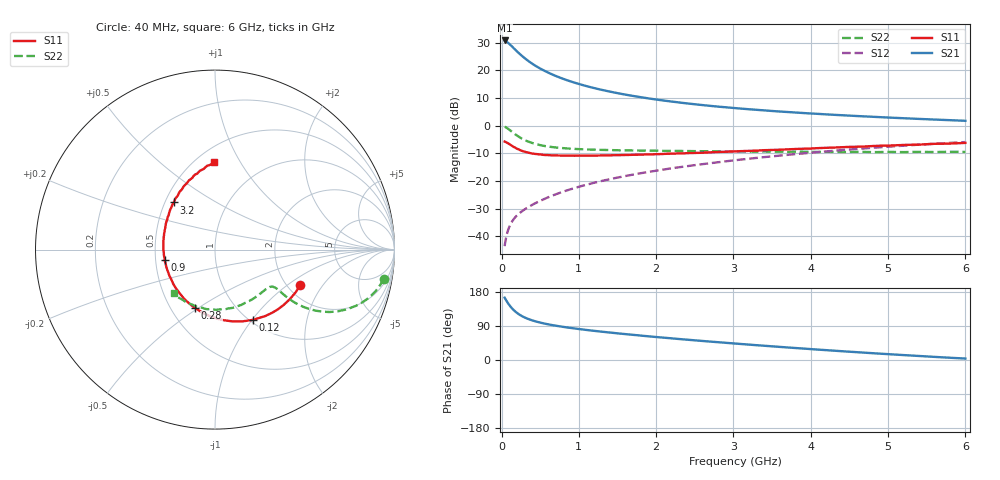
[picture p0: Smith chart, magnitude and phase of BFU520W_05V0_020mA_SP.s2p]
! Filename:  P:\Prog\Test\Noise\ATS_data\Testdata_Net\Run2\BFU520W_APM2013_06_A05_05p0V_020mA_SP_CM01_D.s2p
! Date/Time: Tue 26/Mar/2013 18:01:41
! BFU520W_APM2013_06_A05_05p0V_1to20mA_SP_CM01_Bias8_R.s2p
! MDIF S-parameter v. bias file
! BFU520W_APM2013_06_A05_05p0V_1to20mA_SP_CM01
! Date/time Thu Mar 21 14:22:37 2013
! VAR V_out= 5.0010
! VAR I_out= 19.9950
! VAR V_in= 0.8452
! VAR I_in= 0.2325
! Device data file deembeded for feedlines and parallel
! Original file: \Run2\BFU520W_APM2013_06_A05_05p0V_020mA_SP_CM01_R.s2p
! Feed-files: PR019V01_070313_Feed1.s2p, PR019V01_070313_Feed2.s2p
! Parallel-file: PR019V01_070313_Par.s2p
# MHz S MA R 50
!  Freq-MHz  S11-mag  S11-arg  S21-mag  S21-arg  S12-mag  S12-arg  S22-mag  S22-arg
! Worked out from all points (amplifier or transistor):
!   98 points, 40 MHz to 6 GHz, reference 50 ohm
!   highest |S21| = 30.8 dB at 40 MHz (marker M1)
!   |S21| within 3 dB of that: start of sweep to 164.9 MHz
!   unconditionally stable (mu >= 1): 975.5 MHz to 2.09 GHz
!   at 300 MHz: K = 0.71, MSG = 27.4 dB, |S12| = -30.3 dB
!   at 1.6 GHz: K = 1.01, MAG = 14.0 dB, |S12| = -18.3 dB
!   at 6 GHz: K = 0.84, MSG = 3.8 dB, |S12| = -5.9 dB
!   S11 on the Smith chart (normalised r, x): 40 MHz: 2.33, -1.26; 120 MHz: 1.04, -1.01; 280 MHz: 0.66, -0.49; 900 MHz: 0.56, -0.07; 3.2 GHz: 0.56, +0.33; 6 GHz: 0.61, +0.78
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40  0.5154 -22.7  34.82 164.6  0.006581 81.1  0.955 -9.9
50  0.5081 -28.1  34.44 161.0  0.008026 79.9  0.9415 -12.1
60  0.5002 -33.4  33.41 157.6  0.009551 78.1  0.925 -14.4
80  0.4831 -43.6  31.92 151.1  0.01223 75.0  0.8875 -18.4
100  0.4641 -52.8  30.16 145.3  0.01463 72.4  0.8456 -21.7
120  0.4451 -61.6  28.48 140.0  0.01681 70.4  0.8045 -24.5
160  0.4109 -76.6  25.04 131.3  0.02055 67.7  0.7273 -28.6
200  0.3831 -89.1  22.08 124.4  0.02372 66.3  0.6616 -31.0
240  0.3608 -99.7  19.62 118.7  0.02653 65.9  0.6088 -32.5
280  0.344 -108.7  17.54 114.2  0.02924 65.9  0.5665 -33.2
380  0.3167 -126.1  13.73 105.8  0.0357 67.0  0.4939 -33.6
500  0.3007 -140.8  10.81 98.8  0.04353 68.8  0.4444 -33.0
700  0.2888 -157.2  7.949 90.5  0.05707 71.0  0.4026 -32.4
900  0.2859 -168.6  6.277 84.5  0.07101 72.2  0.3824 -32.7
1050  0.286 -175.4  5.426 80.5  0.08175 72.7  0.3736 -33.6
1500  0.2917 168.7  3.876 70.3  0.1148 72.5  0.359 -38.2
2050  0.3052 154.5  2.905 59.8  0.1568 70.7  0.3508 -45.9
3100  0.3457 133.0  2.032 42.2  0.2432 64.8  0.3413 -64.7
3200  0.3492 131.2  1.981 40.6  0.2519 64.2  0.3399 -66.6
4100  0.3921 116.6  1.631 27.3  0.3326 57.1  0.3343 -86.0
5200  0.4474 100.8  1.362 13.0  0.434 46.8  0.3317 -112.3
6000  0.4874 90.4  1.224 3.8  0.5045 38.4  0.3342 -133.3
